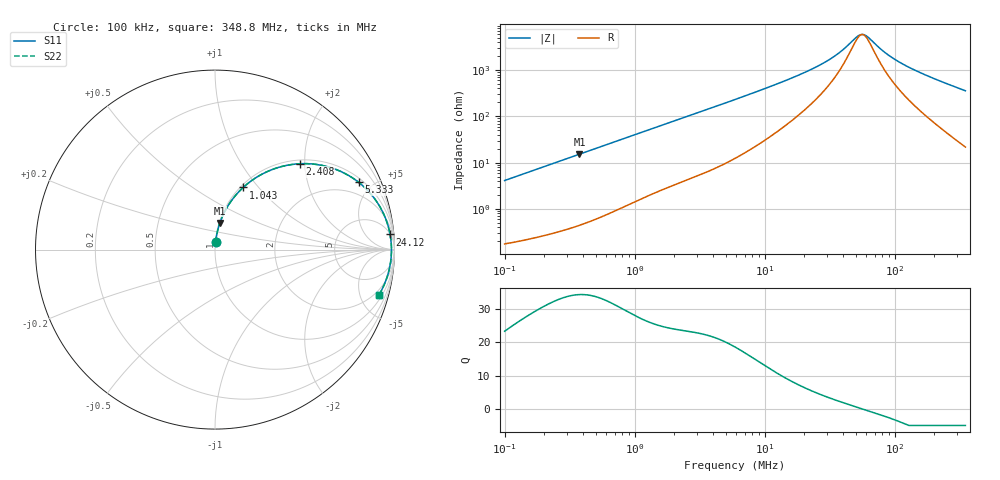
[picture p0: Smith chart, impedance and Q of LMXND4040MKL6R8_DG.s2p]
! LMXND4040MKL6R8_DG  S-PARAMETER MODEL  ( General Type )
! Model Generated by TAIYO YUDEN Corporation (http://www.ty-top.com)
! Version 1.0
! TAIYO YUDEN Control No. 191023NI43SB-FBB
! Copyright(c) 2019 TAIYO YUDEN CO.,LTD. All Rights Reserved.
! Product Description (link to TY-COMPAS)
! https://ds.yuden.co.jp/TYCOMPAS/or/detail?pn=LMXND4040MKL6R8MDG&u=M
! Products Name : Inductors
! Characteristics :
!  Inductance : 6.8 uH , SRF(min) : 35 MHz , DC Resistance(max) : 0.15 Ohm
!  Rated Current : Saturation :900 mA , Temp Rise : 1300 mA
!  Case Size : 4.0 x 4.0 / 0.157 x 0.157 [mm/inch] , Thickness : 1.2 / 0.047 [mm/inch]
!  (Conditions: Temperature = 25 degC , DC Bias Current/Voltage = 0A / 0V)
! External Node Assignments :
!  1  o---GGG---o  2
! GND o---------o GND
! Frequency Range : 0.1MHz  -  348.750116MHz  [ 402 STEP ]
# MHz S RI R 50
! Freq[MHz].  S11 Real  S11 Imag  S21 Real  S21 Imag  S12 Real  S12 Imag  S22 Real  S22 Imag
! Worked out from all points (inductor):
!   401 points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, 100 kHz to 348.8 MHz, reference 50 ohm
!   read as one part in series: L = 6.53 uH near 104.2 kHz
!   highest Q = 34.4 at 376.4 kHz (marker M1), where L = 6.46 uH
!   self-resonance near 56.15 MHz
!   S11 on the Smith chart (normalised r, x): 100 kHz: 1.00, +0.08; 1.043 MHz: 1.03, +0.83; 2.408 MHz: 1.08, +1.89; 5.333 MHz: 1.21, +4.16; 24.12 MHz: 5, +22; 348.8 MHz: 1.43, -7.13
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0.1  0.00344 0.0409  0.9966 -0.0409  0.9966 -0.0409  0.00344 0.0409
0.20416  0.00952 0.0823  0.9905 -0.0823  0.9905 -0.0823  0.00952 0.0823
0.376408  0.0269 0.1479  0.9731 -0.1479  0.9731 -0.1479  0.0269 0.1479
0.392077  0.0289 0.1537  0.9711 -0.1537  0.9711 -0.1537  0.0289 0.1537
0.666246  0.074 0.2465  0.926 -0.2465  0.926 -0.2465  0.074 0.2465
1.043453  0.1571 0.3463  0.8429 -0.3463  0.8429 -0.3463  0.1571 0.3463
1.537242  0.2785 0.4288  0.7215 -0.4288  0.7215 -0.4288  0.2785 0.4288
2.407579  0.4726 0.4785  0.5274 -0.4785  0.5274 -0.4785  0.4726 0.4785
3.475312  0.6417 0.4577  0.3583 -0.4577  0.3583 -0.4577  0.6417 0.4577
5.333051  0.8004 0.375  0.1996 -0.375  0.1996 -0.375  0.8004 0.375
5.905507  0.8289 0.3507  0.1711 -0.3507  0.1711 -0.3507  0.8289 0.3507
10.45281  0.93 0.2184  0.07 -0.2184  0.07 -0.2184  0.93 0.2184
23.15412  0.9748 0.0891  0.0252 -0.0891  0.0252 -0.0891  0.9748 0.0891
24.11798  0.9757 0.0841  0.0243 -0.0841  0.0243 -0.0841  0.9757 0.0841
34.81401  0.9812 0.0443  0.0188 -0.0443  0.0188 -0.0443  0.9812 0.0443
50.2536  0.9831 0.00993  0.0169 -0.00993  0.0169 -0.00993  0.9831 0.00993
55.64788  0.9833 0.000803  0.0167 -0.000803  0.0167 -0.000803  0.9833 0.000803
61.62119  0.9832 -0.00832  0.0168 0.00832  0.0168 0.00832  0.9832 -0.00832
90.78195  0.9813 -0.0445  0.0187 0.0445  0.0187 0.0445  0.9813 -0.0445
115.9511  0.9783 -0.0703  0.0217 0.0703  0.0217 0.0703  0.9783 -0.0703
154.2634  0.9719 -0.1053  0.0281 0.1053  0.0281 0.1053  0.9719 -0.1053
348.7501  0.9141 -0.2513  0.0859 0.2513  0.0859 0.2513  0.9141 -0.2513
